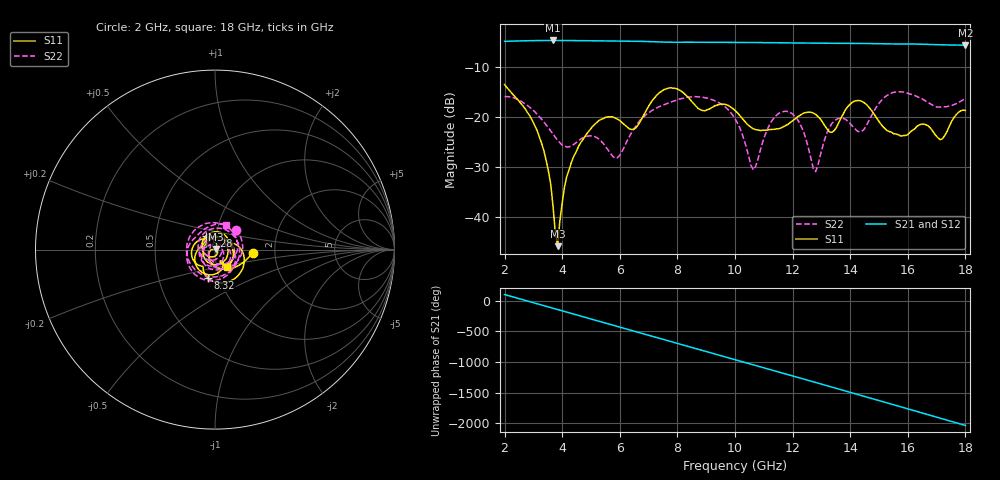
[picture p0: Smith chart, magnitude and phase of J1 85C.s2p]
!Agilent Technologies,E8363B,SG43030131,A.07.50.48
!Agilent E8363B: A.07.50.48
!Date: Wednesday, December 17, 2025 22:39:13
!Correction: S11(Full 2 Port(1,2))
!S21(Full 2 Port(1,2))
!S12(Full 2 Port(1,2))
!S22(Full 2 Port(1,2))
!S2P File: Measurements: S11, S21, S12, S22:
# Hz S  dB  R 50
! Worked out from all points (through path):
!   201 points, 2 GHz to 18 GHz, reference 50 ohm
!   highest |S21| = -4.66 dB at 3.68 GHz (marker M1); lowest = -5.6 dB at 18 GHz (marker M2)
!   group delay of S21, straight-line fit = 370 ps
!   lowest |S11| = -46.0 dB at 3.84 GHz (marker M3), VSWR 1.01, Z = 50.3 + j0.402 ohm
!   |S11| at or under -10 dB: start of sweep to end of sweep
!   |S22| runs from -31.0 to -14.9 dB; largest |S21 - S12| = 0.0022
!   S11 on the Smith chart (normalised r, x): 2 GHz: 1.53, -0.05; 5.28 GHz: 0.90, +0.14; 8.32 GHz: 0.88, -0.29; 18 GHz: 1.12, -0.22
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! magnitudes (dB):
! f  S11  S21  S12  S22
! 2 GHz  -13.5  -4.8  -4.8  -15.9
! 3.12 GHz  -22.6  -4.7  -4.7  -19.4
! 3.44 GHz  -28.7  -4.7  -4.7  -21.6
! 3.68 GHz  -37.8  -4.7  -4.7  -23.4
! 3.84 GHz  -46.0  -4.7  -4.7  -24.7
! 4.16 GHz  -31.9  -4.7  -4.7  -26.0
! 4.72 GHz  -24.5  -4.7  -4.7  -24.2
! 5.28 GHz  -20.7  -4.7  -4.7  -24.5
! 5.92 GHz  -20.4  -4.8  -4.8  -28.2
! 6.48 GHz  -22.5  -4.8  -4.8  -22.5
! 7.36 GHz  -15.2  -5.0  -5.0  -18.0
! 8.32 GHz  -15.8  -5.0  -5.0  -16.1
! 10 GHz  -18.7  -5.1  -5.1  -20.3
! 10.64 GHz  -22.4  -5.1  -5.1  -30.7
! 11.28 GHz  -22.5  -5.1  -5.1  -20.8
! 12 GHz  -20.8  -5.2  -5.2  -19.4
! 12.72 GHz  -19.2  -5.2  -5.2  -30.4
! 13.44 GHz  -22.8  -5.2  -5.2  -20.9
! 14.32 GHz  -16.7  -5.2  -5.2  -23.0
! 15.36 GHz  -23.0  -5.4  -5.4  -15.4
! 17.12 GHz  -24.6  -5.5  -5.5  -18.0
! 18 GHz  -18.7  -5.6  -5.6  -16.3
